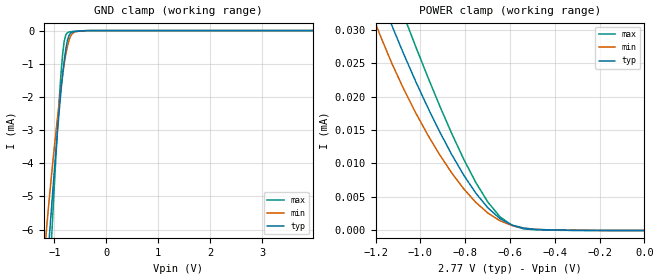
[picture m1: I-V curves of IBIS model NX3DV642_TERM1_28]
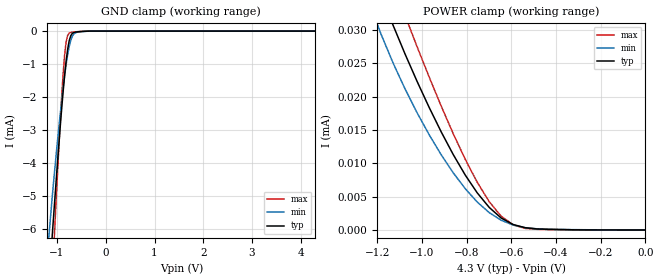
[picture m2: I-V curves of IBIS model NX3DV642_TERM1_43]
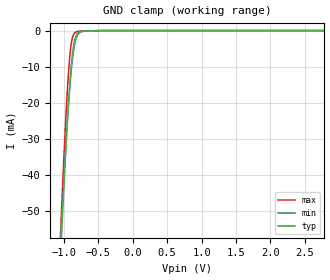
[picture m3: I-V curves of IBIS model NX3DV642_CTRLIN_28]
| NXP Semiconductors
| Logic Products Group
| IBIS model of NX3DV642
| 3-LANE HIGH-SPEED MIPI COMPATIBLE SWITCH
|[Packages]:
|[Package1]: XQFN24 (GU) 24-pins Package
[IBIS Ver]   3.2
[File Name]   nx3dv642.ibs
[File Rev]   1.0
[Date]   27-Jul-2012
[Source]   File created from simulations by LPG
   NXP Semiconductors Nijmegen
[Notes]   V1.0   Ibis model.
   Revision History
   Version Date   Author/ Description
   Editor
   1.0   July 2012   RRV   Initial Model
   Remarks: - The Power Clamp curves have been omitted from the input
   since the is no power clamp diode.
   - IBISCHK 5.0.3 used
   - Following notes/warnings are caused by normal switch behaviour:
   'Series_MOSFET has Decreasing Current'
   'Series_MOSFET data is non-monotonic'
[Disclaimer]
   NXP Semiconductors warrants and represents that the IBIS model
   identified herein is owned by NXP Semiconductors (NXP). The
   model provided is not warranted as fully representing all of the
   operating characteristics and specifications of the semiconductor
   products to which the model relates.  Moreover, unless there is a
   signed, written agreement to the contrary, this IBIS model is
   furnished on an "as is" basis without support or warranty of any
   kind, either expressed or implied, regarding the use thereof, and
   NXP specifically disclaims all implied warranties of
   merchantability and fitness of the model for any purpose.
   NXP does not assume any liability arising out of the application
   or use of this IBIS model including infringement of patents and
   copyrights, nor does NXP convey any license under its patents and
   copyrights or the rights of others.
   NXP provides IBIS models as a service to our customers. You and
   your company shall not distribute, convey, sell, or give these models
   to anyone else without receiving prior written permission from
   NXP.
   NXP reserves the right to make changes without notice to these
   IBIS models to improve reliability, function, or design.
   Please be aware that your receipt and subsequent use of the IBIS
   information provided shall serve as acceptance of the terms and
   conditions of this agreement.  If you do not accept these terms,
   you should return or destroy the IBIS models and any other
   accompanying information immediately.
[Copyright]
   (C) Copyright 2012 NXP Semiconductors
   All rights reserved
|   Info for  XQFN24 (GU) 24-pins Package
[Component]   NX3DV642_GU
[Manufacturer]   NXP Semiconductors
[Package]
|   Typ   Min   Max
R_pkg   7.178E-02   7.385E-04   1.082E-01
L_pkg   9.170E-10   5.893E-12   1.383E-09
C_pkg   1.612E-13   7.814E-14   2.021E-13
[Pin] signal_name   model_name   R_pin   L_pin   C_pin
   1   CLKP   NX3DV642_TERM1 7.487E-02 9.566E-10 1.679E-13
   2   CLKM   NX3DV642_TERM1 6.173E-02 7.876E-10 1.527E-13
   3   1DP   NX3DV642_TERM1 5.272E-02 6.748E-10 1.429E-13
   4   1DM   NX3DV642_TERM1 5.343E-02 6.814E-10 1.392E-13
   5   2DP   NX3DV642_TERM1 6.100E-02 7.808E-10 1.525E-13
   6   2DM   NX3DV642_TERM1 7.520E-02 9.603E-10 1.682E-13
   7   NC   NC 7.952E-04 8.977E-12 8.315E-14
   8   OEN   NX3DV642_CTRLIN 9.011E-02 1.152E-09 1.813E-13
   9   GND   GND 9.260E-02 1.184E-09 1.841E-13
   10   VCC   POWER 9.766E-02 1.248E-09 1.900E-13
   11   S   NX3DV642_CTRLIN 1.082E-01 1.383E-09 2.021E-13
   12   2D1M   NX3DV642_TERM1 1.003E-01 1.283E-09 1.931E-13
   13   2D1P   NX3DV642_TERM1 8.172E-02 1.044E-09 1.716E-13
   14   1D1M   NX3DV642_TERM1 6.702E-02 8.556E-10 1.546E-13
   15   1D1P   NX3DV642_TERM1 5.939E-02 7.578E-10 1.458E-13
   16   CLK1M   NX3DV642_TERM1 5.180E-02 6.605E-10 1.371E-13
   17   CLK1P   NX3DV642_TERM1 5.486E-02 6.997E-10 1.406E-13
   18   2D2M   NX3DV642_TERM1 6.990E-02 8.926E-10 1.579E-13
   19   2D2P   NX3DV642_TERM1 1.042E-01 1.332E-09 1.975E-13
   20   1D2M   NX3DV642_TERM1 9.490E-02 1.213E-09 1.868E-13
   21   1D2P   NX3DV642_TERM1 9.215E-02 1.178E-09 1.836E-13
   22   CLK2M   NX3DV642_TERM1 8.833E-02 1.129E-09 1.792E-13
   23   CLK2P   NX3DV642_TERM1 8.912E-02 1.139E-09 1.801E-13
   24   NC   NC 7.385E-04 5.893E-12 7.814E-14
[Series Pin Mapping]  pin_2  model_name   function_table_group
1   17   NX3DV642_SWITCH1   1
1   22   NX3DV642_SWITCH1   2
17   1   NX3DV642_SWITCH1   3
22   1   NX3DV642_SWITCH1   4
2   16   NX3DV642_SWITCH1   1
2   23   NX3DV642_SWITCH1   2
16   2   NX3DV642_SWITCH1   3
23   2   NX3DV642_SWITCH1   4
3   15   NX3DV642_SWITCH1   1
3   20   NX3DV642_SWITCH1   2
15   3   NX3DV642_SWITCH1   3
20   3   NX3DV642_SWITCH1   4
4   14   NX3DV642_SWITCH1   1
4   21   NX3DV642_SWITCH1   2
14   4   NX3DV642_SWITCH1   3
21   4   NX3DV642_SWITCH1   4
5   13   NX3DV642_SWITCH1   1
5   19   NX3DV642_SWITCH1   2
13   5   NX3DV642_SWITCH1   3
19   5   NX3DV642_SWITCH1   4
6   12   NX3DV642_SWITCH1   1
6   18   NX3DV642_SWITCH1   2
12   6   NX3DV642_SWITCH1   3
18   6   NX3DV642_SWITCH1   4
[Series Switch Groups]
| Function Group States
On 1 /   | Common CLK/D to independent CLK1/D1, S=Low,  En=Low
On 2 /   | Common CLK/D to independent CLK2/D2, S=High, En=Low
On 3 /   | Independent CLK1/D1 to common CLK/D, S=Low,  En=Low
On 4 /   | Independent CLK1/D1 to common CLK/D, S=High, En=Low
Off 1 2 3 4 /   | En=High
[Model Selector]   NX3DV642_SWITCH1
NX3DV642_SWITCH1_28   3.3V-Vcc Series switch model
NX3DV642_SWITCH1_43   4.3V-Vcc Series switch model
[Model Selector]   NX3DV642_TERM1
NX3DV642_TERM1_28   2.775V-Vcc Series Switch I/O model
NX3DV642_TERM1_43   4.3V-Vcc Series Switch I/O model
[Model Selector]   NX3DV642_CTRLIN
NX3DV642_CTRLIN_28   2.775V-Vcc input model
NX3DV642_CTRLIN_43   4.3V-Vcc input model
|   Model NX3DV642_SWITCH1_28
[Model]   NX3DV642_SWITCH1_28
Model_type   Series_switch
C_comp   8.012pF   7.587pF   8.348pF
| ON capacitance of switch
|Ambient temperature:   25   85   -40
[Temperature Range]   30   90   -35
[Voltage Range]   2.775   2.65   2.775
[Off]
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[On]
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|   Model NX3DV642_SWITCH1_43
[Model]   NX3DV642_SWITCH1_43
Model_type   Series_switch
C_comp   8.012pF   7.587pF   8.348pF
| ON capacitance of switch
|Ambient temperature:   25   85   -40
[Temperature Range]   30   90   -35
[Voltage Range]   4.3   4.3   4.3
[Off]
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[On]
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| Models and submodels in the file (6): NX3DV642_TERM1_28 (Terminator), NX3DV642_SWITCH1_28 (Series_switch), NX3DV642_TERM1_43 (Terminator), NX3DV642_SWITCH1_43 (Series_switch), NX3DV642_CTRLIN_28 (Input), NX3DV642_CTRLIN_43 (Input)
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| Remark: If your software does not support the Model Selector
|   Please comment out the lines of the Model Selector, which
|   contain the name of the Model, except the one you want to use.
|   Model NX3DV642_TERM1_28
[Model]   NX3DV642_TERM1_28
Model_type   Terminator
C_comp   8.012pF   7.587pF   8.348pF
| ON capacitance of switch
|Ambient temperature:   25   85   -40
[Temperature Range]   30   90   -35
[Voltage Range]   2.775   2.65   2.775
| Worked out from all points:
|   GND clamp passes 1 mA (typ) near -0.82 V on its own axis
|   POWER clamp passes 1 mA (typ) near -2.67 V on its own axis
|Process Range   nominal   slow   fast
[GND_clamp]
|   voltage   I(typ)   I(min)   I(max)
-4.3V     -2.17A     -1.847A    -2.547A
-1.156V   -7.48mA    -6.066mA   -9.367mA
-1.094V   -6.137mA   -4.981mA   -7.446mA
-1.062V   -5.482mA   -4.469mA   -6.496mA
-1.031V   -4.837mA   -3.975mA   -5.558mA
-906.2mV  -2.404mA   -2.15mA    -2.064mA
-843.8mV  -1.356mA   -1.361mA   -740.6uA
-812.5mV  -915.8uA   -1.017mA   -332.5uA
-750mV    -299uA     -474.7uA   -62.81uA
-656.2mV  -44.73uA   -91.84uA   -27.59uA
-406.2mV  -4.726uA   -7.593uA   -1.957uA
4.3V      0A         0A         0A
[POWER_clamp]
|   voltage   I(typ)   I(min)   I(max)
-4.3V     3.367mA    2.572mA    4.722mA
-1.236V   40.39uA    34.19uA    46.96uA
-1.183V   35.35uA    29.36uA    41.88uA
-1.129V   30.72uA    25.05uA    36.95uA
-1.075V   26.38uA    21.15uA    32.16uA
-1.021V   22.28uA    17.58uA    27.48uA
-913.7mV  14.73uA    11.3uA     18.6uA
-806.3mV  8.25uA     6.205uA    10.62uA
-698.7mV  3.384uA    2.603uA    4.238uA
-645mV    1.786uA    1.455uA    2.054uA
-537.5mV  334.4nA    347.5nA    232.6nA
0V        64.42pA    71.44pA    73.44pA
|   Model NX3DV642_TERM1_43
[Model]   NX3DV642_TERM1_43
Model_type   Terminator
C_comp   8.012pF   7.587pF   8.348pF
| ON capacitance of switch
|Ambient temperature:   25   85   -40
[Temperature Range]   30   90   -35
[Voltage Range]   4.3   4.3   4.3
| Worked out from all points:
|   GND clamp passes 1 mA (typ) near -0.82 V on its own axis
|   POWER clamp passes 1 mA (typ) near -2.67 V on its own axis
|Process Range   nominal   slow   fast
[GND_clamp]
|   voltage   I(typ)   I(min)   I(max)
-4.3V     -2.17A     -1.847A    -2.547A
-1.156V   -7.48mA    -6.066mA   -9.367mA
-1.094V   -6.137mA   -4.981mA   -7.446mA
-1.062V   -5.482mA   -4.469mA   -6.496mA
-1.031V   -4.837mA   -3.975mA   -5.558mA
-906.2mV  -2.404mA   -2.15mA    -2.064mA
-843.8mV  -1.356mA   -1.361mA   -740.6uA
-812.5mV  -915.8uA   -1.017mA   -332.5uA
-750mV    -299uA     -474.7uA   -62.81uA
-656.2mV  -44.73uA   -91.84uA   -27.59uA
-406.2mV  -4.726uA   -7.593uA   -1.957uA
4.3V      0A         0A         0A
[POWER_clamp]
|   voltage   I(typ)   I(min)   I(max)
-4.3V     3.367mA    2.572mA    4.722mA
-1.236V   40.39uA    34.19uA    46.96uA
-1.183V   35.35uA    29.36uA    41.88uA
-1.129V   30.72uA    25.05uA    36.95uA
-1.075V   26.38uA    21.15uA    32.16uA
-1.021V   22.28uA    17.58uA    27.48uA
-913.7mV  14.73uA    11.3uA     18.6uA
-806.3mV  8.25uA     6.205uA    10.62uA
-698.7mV  3.384uA    2.603uA    4.238uA
-645mV    1.786uA    1.455uA    2.054uA
-537.5mV  334.4nA    347.5nA    232.6nA
0V        64.42pA    71.44pA    73.44pA
|   Model NX3DV642_CTRLIN_28
[Model]   NX3DV642_CTRLIN_28
Model_type   Input
Vinl = 0.5V
Vinh = 1.3V
C_comp   0.867pF   0.821pF   0.937pF
[Model Spec]
| Note: The input and output voltage ratings may be exceeded if the input and
|   output current ratings are observed (please refer to the data sheet)
|   Subparameter   typ   min   max
| Thresholds
Vinl   0.5   0.5   0.5
Vinh   1.3   1.3   1.3
| Overshoot
S_overshoot_high   2.775   2.775   2.775
S_overshoot_low   -0.5   -0.5   -0.5
D_overshoot_high   5.5   5.5   5.5
D_overshoot_low   -0.95   -0.9   -1.0
D_overshoot_time   3n   3n   3n
|Ambient temperature:   25   85   -40
[Temperature Range]   30   90   -35
[Voltage Range]   2.775   2.65   2.775
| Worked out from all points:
|   GND clamp passes 1 mA (typ) near -0.81 V on its own axis
|Process Range   nominal   slow   fast
[GND_clamp]
|   voltage   I(typ)   I(min)   I(max)
-2.775V   -852mA     -780.4mA   -921.4mA
-1.062V   -67.87mA   -63.41mA   -61.74mA
-1.047V   -61.37mA   -57.56mA   -54.65mA
-1.031V   -55mA      -51.83mA   -47.72mA
-968.8mV  -31.2mA    -30.51mA   -22.4mA
-921.9mV  -16.31mA   -17.15mA   -8.299mA
-906.2mV  -12.27mA   -13.45mA   -5.215mA
-875mV    -6.075mA   -7.52mA    -1.726mA
-828.1mV  -1.58mA    -2.478mA   -380.1uA
-765.6mV  -318.6uA   -493.1uA   -167.8uA
-656.2mV  -116.7uA   -110uA     -82.08uA
2.775V    0A         0A         0A
